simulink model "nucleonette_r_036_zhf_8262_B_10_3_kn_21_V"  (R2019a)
settings: Solver=VariableStepAuto  StartTime=0.0  StopTime=727544.216  FixedStep=0.2  RelTol=1e-6
libraries: simulink x6
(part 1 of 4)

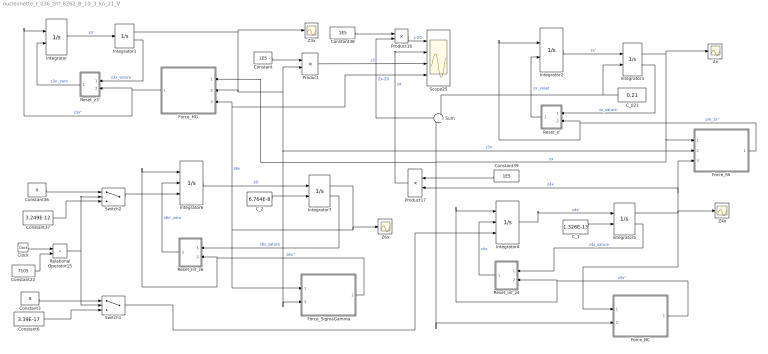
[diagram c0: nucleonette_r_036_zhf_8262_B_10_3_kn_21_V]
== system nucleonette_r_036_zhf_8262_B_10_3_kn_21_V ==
  C_021 : Constant  Value=0.21
  C_1 : Constant  Value=1.326E-13
  C_2 : Constant  Value=6.764E-8
  Clock : Clock
  Constant : Constant  Value=1E5
  Constant22 : Constant  Value=7105
  Constant3 : Constant  Value=0
  Constant36 : Constant  Value=0
  Constant37 : Constant  Value=3.249E-12
  Constant38 : Constant  Value=1E5
  Constant39 : Constant  Value=1E5
  Constant6 : Constant  Value=3.39E-17
  Force_BC : Subsystem
  Force_FA : Subsystem
  Force_HG : Subsystem
  Force_SigmaGamma : Subsystem
  Integrator : Integrator  ExternalReset=level
  Integrator1 : Integrator  LimitOutput=on  UpperSaturationLimit=0  LowerSaturationLimit=-1.80E-12  ShowSaturationPort=on  ZeroCross=off
  Integrator2 : Integrator  ExternalReset=level
  Integrator3 : Integrator  InitialConditionSource=external  LimitOutput=on  UpperSaturationLimit=0.21000000000316  LowerSaturationLimit=0.21  ShowSaturationPort=on
  Integrator4 : Integrator  ExternalReset=level  InitialConditionSource=external  AbsoluteTolerance=1E-22
  Integrator5 : Integrator  InitialConditionSource=external  LimitOutput=on  LowerSaturationLimit=0  ShowSaturationPort=on  ZeroCross=off
  Integrator6 : Integrator  ExternalReset=level  InitialConditionSource=external
  Integrator7 : Integrator  InitialConditionSource=external  LimitOutput=on  LowerSaturationLimit=0.0  ShowSaturationPort=on  ZeroCross=off
  Product : Product
  Product16 : Product
  Product17 : Product
  Relational Operator15 : RelationalOperator  Operator=>  OutDataTypeStr=boolean  RndMeth=Simplest
  Reset_Inf_z4 : Subsystem
  Reset_Inf_z6 : Subsystem
  Reset_z' : Subsystem
  Reset_z3' : Subsystem
  Scope25 : Scope  NumInputPorts=4
  Sum : Sum  Inputs=-+
  Switch1 : Switch  Criteria=u2 > Threshold
  Switch2 : Switch  Criteria=u2 > Threshold
  Z3x : Scope
  Z4x : Scope
  Z6x : Scope
  Zx : Scope
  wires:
  Integrator1/1 -> Z3x/1, Product/2, Force_FA/2(In2), Force_SigmaGamma/2(In2), Force_HG/2(In2)  "z3x"
  Integrator3/1 -> Force_HG/1(In1), Force_BC/2(In2), Sum/2, Force_FA/1(In1), Zx/1  "zx"
  C_021/1 -> Sum/1, Integrator3/2
  Force_FA/1(Out1) -> Integrator2/1, Reset_z'/2(In3)  "pre_zx''"
  Integrator3/2 -> Reset_z'/1(In1)  "zx_sature"
  Integrator2/1 -> Integrator3/1  "zx'"
  Force_HG/1(Out1) -> Integrator/1, Reset_z3'/2(In3)  "z3x''"
  Sum/1 -> Product16/2  "Zx-Z0"
  C_1/1 -> Integrator5/2
  Integrator5/2 -> Reset_Inf_z4/1(In1)  "z4x_sature"
  Integrator5/1 -> Product17/2, Force_FA/3(In3), Z4x/1, Force_BC/1(In1)  "z4x"
  Integrator7/2 -> Reset_Inf_z6/1(In1)  "z6x_sature"
  Reset_Inf_z6/1(Out1) -> Integrator6/2  "z6x'_zero"
  Integrator7/1 -> Z6x/1, Force_SigmaGamma/1(In1), Scope25/4, Force_HG/3(In3)  "z6x"
  Force_SigmaGamma/1(Out1) -> Reset_Inf_z6/2(In3), Integrator6/1  "z6x''"
  C_2/1 -> Integrator7/2
  Reset_z'/1(Out1) -> Integrator2/2  "zx'_reset"
  Integrator1/2 -> Reset_z3'/1(In1)  "z3x_sature"
  Reset_z3'/1(Out1) -> Integrator/2  "z3x'_zero"
  Integrator6/1 -> Integrator7/1  "z6'"
  Integrator4/1 -> Integrator5/1  "z4x'"
  Reset_Inf_z4/1(Out1) -> Integrator4/2  "z4x"
  Constant22/1 -> Relational Operator15/2
  Clock/1 -> Relational Operator15/1
  Constant6/1 -> Switch1/3
  Force_BC/1(Out1) -> Integrator4/1, Reset_Inf_z4/2(In3)  "z4x''"
  Switch1/1 -> Integrator4/3
  Constant3/1 -> Switch1/1
  Integrator/1 -> Integrator1/1  "z3'"
  Product/1 -> Scope25/3  "z3"
  Constant/1 -> Product/1
  Constant37/1 -> Switch2/3
  Constant36/1 -> Switch2/1
  Switch2/1 -> Integrator6/3
  Relational Operator15/1 -> Switch1/2, Switch2/2
  Product16/1 -> Scope25/1  "z-Z0"
  Constant38/1 -> Product16/1
  Constant39/1 -> Product17/1
  Product17/1 -> Scope25/2  "z4"

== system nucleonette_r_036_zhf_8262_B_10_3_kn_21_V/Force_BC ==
  In1 : Inport
  In2 : Inport  Port=2
  Add26 : Sum  Inputs=-++
  Constant23 : Constant  Value=3.16E-12
  F_BA : Subsystem
  F_BD : Subsystem
  F_BE : Subsystem
  F_BF : Subsystem
  F_CA : Subsystem
  F_CD : Subsystem
  F_CE : Subsystem
  F_CF : Subsystem
  Scope14 : Scope
  Sum1 : Sum  Inputs=|-|+|-|+|+|-|+|-
  Z0_1 : Constant  Value=0.21
  Out1 : Outport
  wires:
  Sum1/1 -> Scope14/1, Out1/1  "pre_z4x''"
  In1/1 -> F_CE/1(In1), F_BD/1(In1), F_CD/1(In1), F_CF/1(In1), F_CA/1(In1), F_BA/1(In1), F_BF/1(In1), F_BE/1(In1)  "z4"
  F_BF/1(Out1) -> Sum1/5
  F_BE/1(Out1) -> Sum1/1
  Z0_1/1 -> Add26/2  "Z0"
  In2/1 -> Add26/1  "z"
  Add26/1 -> F_CA/2(In2), F_BA/2(In2), F_CF/2(In2), F_BF/2(In2)  "z0 - z + delta"
  F_CE/1(Out1) -> Sum1/2
  F_BD/1(Out1) -> Sum1/3
  F_CD/1(Out1) -> Sum1/4
  F_CA/1(Out1) -> Sum1/8
  F_BA/1(Out1) -> Sum1/7
  Constant23/1 -> Add26/3  "Delta_1"
  F_CF/1(Out1) -> Sum1/6  "ncf/dcf_3"

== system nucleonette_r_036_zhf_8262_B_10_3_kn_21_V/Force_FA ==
  In1 : Inport
  In2 : Inport  Port=2
  In3 : Inport  Port=3
  Add1 : Sum  Inputs=-++
  Add26 : Sum  Inputs=-+
  Delta : Constant  Value=3.16E-12
  F_AB : Subsystem
  F_AC : Subsystem
  F_AD : Subsystem
  F_AE : Subsystem
  F_AG : Subsystem
  F_AH : Subsystem
  F_AI : Subsystem
  F_AJ : Subsystem
  F_FB : Subsystem
  F_FC : Subsystem
  F_FD : Subsystem
  F_FE : Subsystem
  F_FG : Subsystem
  F_FH : Subsystem
  F_FI : Subsystem
  F_FJ : Subsystem
  Scope1 : Scope
  Sum : Sum  Inputs=|++
  Sum1 : Sum  Inputs=|+|-|+|-|-|+|-|+
  Sum2 : Sum  Inputs=|-|+|+|-|-|+|+|-
  Z0_1 : Constant  Value=0.21
  Z0_2 : Constant  Value=0.21
  Out1 : Outport
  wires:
  Sum1/1 -> Sum/1  "pre_zx''_1"
  In1/1 -> F_AI/1(In1), F_AJ/1(In1), F_AG/1(In1), Add1/1, F_AH/1(In1), F_FH/1(In1), F_FG/1(In1), F_FJ/1(In1), F_FI/1(In1)
  F_FG/1(Out1) -> Sum1/5
  F_FI/1(Out1) -> Sum1/1
  Z0_1/1 -> Add26/2  "Z0"
  In2/1 -> Add26/1  "z3"
  Add26/1 -> F_FH/2(In2), F_AG/2(In2), F_FG/2(In2), F_AH/2(In2)  "z0 - z3"
  F_AI/1(Out1) -> Sum1/2
  F_FJ/1(Out1) -> Sum1/3
  F_AJ/1(Out1) -> Sum1/4
  F_AH/1(Out1) -> Sum1/8
  F_FH/1(Out1) -> Sum1/7
  F_AG/1(Out1) -> Sum1/6
  F_AE/1(Out1) -> Sum2/8
  F_FE/1(Out1) -> Sum2/7
  F_AD/1(Out1) -> Sum2/6
  Z0_2/1 -> Add1/2  "Z0"
  F_AC/1(Out1) -> Sum2/4
  F_FC/1(Out1) -> Sum2/3
  F_AB/1(Out1) -> Sum2/2
  Add1/1 -> F_AE/1(In1), F_FE/1(In1), F_AD/1(In1), F_FD/1(In1), F_AC/1(In1), F_FC/1(In1), F_AB/1(In1), F_FB/1(In1)  "z0 - z + delta"
  F_FB/1(Out1) -> Sum2/1
  F_FD/1(Out1) -> Sum2/5
  In3/1 -> F_AB/2(In2), F_FC/2(In2), F_AC/2(In2), F_FD/2(In2), F_AD/2(In2), F_AE/2(In2), F_FE/2(In2), F_FB/2(In2)
  Sum2/1 -> Sum/2  "pre_zx''_2"
  Sum/1 -> Scope1/1, Out1/1  "z3''"
  Delta/1 -> Add1/3  "Delta"

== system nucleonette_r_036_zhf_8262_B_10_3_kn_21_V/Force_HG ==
  In1 : Inport
  In2 : Inport  Port=2
  In3 : Inport  Port=3
  Add1 : Sum
  Add26 : Sum  Inputs=-+
  F_HA : Subsystem
  F_HF : Subsystem
  F_HGamma : Subsystem
  F_HI : Subsystem
  F_HJ : Subsystem
  F_HOmega : Subsystem
  F_HPhi : Subsystem
  F_HSigma : Subsystem
  Scope13 : Scope
  Sum : Sum  Inputs=|+|-|+|-
  Sum1 : Sum  Inputs=|+|+|-|-
  Sum2 : Sum  Inputs=|++
  Z0_1 : Constant  Value=0.21
  delta6 : Constant  Value=1.80E-12
  Out1 : Outport
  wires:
  In1/1 -> F_HJ/1(In1), F_HI/1(In1), F_HF/1(In1), F_HA/1(In1)  "zx"
  Sum/1 -> Sum2/1  "pre_z3x''_1"
  F_HA/1(Out1) -> Sum/1
  F_HF/1(Out1) -> Sum/2
  F_HI/1(Out1) -> Sum/3
  F_HJ/1(Out1) -> Sum/4
  F_HPhi/1(Out1) -> Sum1/3
  F_HOmega/1(Out1) -> Sum1/4
  F_HGamma/1(Out1) -> Sum1/2
  In3/1 -> F_HGamma/1(In1), F_HPhi/1(In1), F_HOmega/1(In1), F_HSigma/1(In1)  "z6x"
  F_HSigma/1(Out1) -> Sum1/1
  Sum1/1 -> Sum2/2  "pre_z3x''_2"
  Sum2/1 -> Scope13/1, Out1/1  "z3''"
  Z0_1/1 -> Add26/2  "Z0"
  In2/1 -> Add1/1, Add26/1  "Z3"
  Add26/1 -> F_HJ/2(In2), F_HI/2(In2), F_HF/2(In2), F_HA/2(In2)  "z0 - z3"
  Add1/1 -> F_HSigma/2(In2), F_HOmega/2(In2), F_HPhi/2(In2), F_HGamma/2(In2)  "z3 + delta6"
  delta6/1 -> Add1/2  "delta6"

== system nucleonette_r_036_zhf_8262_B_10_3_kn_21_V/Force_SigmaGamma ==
  In1 : Inport
  In2 : Inport  Port=2
  Add26 : Sum
  F_GammaG : Subsystem
  F_GammaH : Subsystem
  F_GammaOmega : Subsystem
  F_GammaPhi : Subsystem
  F_SigmaG : Subsystem
  F_SigmaH : Subsystem
  F_SigmaOmega : Subsystem
  F_SigmaPhi : Subsystem
  Scope14 : Scope
  Sum1 : Sum  Inputs=|+|-|+|-|+|-|+|-
  delta6 : Constant  Value=1.80E-12
  Out1 : Outport
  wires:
  Sum1/1 -> Scope14/1, Out1/1  "pre_z6x''"
  In1/1 -> F_SigmaOmega/1(In1), F_GammaOmega/1(In1), F_SigmaPhi/1(In1), F_GammaPhi/1(In1), F_SigmaH/1(In1), F_GammaH/1(In1), F_SigmaG/1(In1), F_GammaG/1(In1)  "z6"
  F_SigmaH/1(Out1) -> Sum1/5
  F_SigmaOmega/1(Out1) -> Sum1/1
  In2/1 -> Add26/1  "z3"
  Add26/1 -> F_GammaG/2(In2), F_SigmaG/2(In2), F_SigmaH/2(In2), F_GammaH/2(In2)  "delta6 + z3"
  F_GammaOmega/1(Out1) -> Sum1/2
  F_SigmaPhi/1(Out1) -> Sum1/3
  F_GammaPhi/1(Out1) -> Sum1/4
  F_GammaG/1(Out1) -> Sum1/8
  F_SigmaG/1(Out1) -> Sum1/7
  F_GammaH/1(Out1) -> Sum1/6
  delta6/1 -> Add26/2  "Delta6_1"

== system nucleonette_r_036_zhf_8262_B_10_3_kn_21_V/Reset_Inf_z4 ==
  In1 : Inport
  In3 : Inport  Port=2
  Compare To Zero : simulink/Logic and Bit Operations/Compare To Zero  relop=<  OutDataTypeStr=boolean
  Constant10 : Constant  Value=0
  Logical Operator1 : Logic  AllPortsSameDT=off  OutDataTypeStr=boolean
  Relational Operator4 : RelationalOperator  Operator=<  OutDataTypeStr=boolean  RndMeth=Simplest
  Out1 : Outport
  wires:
  In1/1 -> Compare To Zero/1  "Saturation"
  Constant10/1 -> Relational Operator4/2
  Compare To Zero/1 -> Logical Operator1/1
  Logical Operator1/1 -> Out1/1
  In3/1 -> Relational Operator4/1  "Acceleration"
  Relational Operator4/1 -> Logical Operator1/2  "ForceFz_>_0"

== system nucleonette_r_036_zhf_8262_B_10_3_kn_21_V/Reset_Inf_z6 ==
  In1 : Inport
  In3 : Inport  Port=2
  Compare To Zero : simulink/Logic and Bit Operations/Compare To Zero  relop=<  OutDataTypeStr=boolean
  Constant10 : Constant  Value=0
  Logical Operator1 : Logic  AllPortsSameDT=off  OutDataTypeStr=boolean
  Relational Operator4 : RelationalOperator  Operator=<  OutDataTypeStr=boolean  RndMeth=Simplest
  Out1 : Outport
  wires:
  In1/1 -> Compare To Zero/1  "Saturation"
  Constant10/1 -> Relational Operator4/2
  Compare To Zero/1 -> Logical Operator1/1
  Logical Operator1/1 -> Out1/1
  In3/1 -> Relational Operator4/1  "Acceleration"
  Relational Operator4/1 -> Logical Operator1/2  "ForceFz_>_0"

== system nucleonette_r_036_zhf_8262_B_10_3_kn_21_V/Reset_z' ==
  In1 : Inport
  In3 : Inport  Port=2
  Compare To Zero : simulink/Logic and Bit Operations/Compare To Zero  relop=>  OutDataTypeStr=boolean
  Compare To Zero1 : simulink/Logic and Bit Operations/Compare To Zero  relop=<  OutDataTypeStr=boolean
  Constant10 : Constant  Value=0
  Logical Operator1 : Logic  AllPortsSameDT=off  OutDataTypeStr=boolean
  Logical Operator2 : Logic  AllPortsSameDT=off  OutDataTypeStr=boolean
  Logical Operator3 : Logic  Operator=OR  AllPortsSameDT=off  OutDataTypeStr=boolean
  Relational Operator1 : RelationalOperator  Operator=<  OutDataTypeStr=boolean  RndMeth=Simplest
  Relational Operator4 : RelationalOperator  Operator=>  OutDataTypeStr=boolean  RndMeth=Simplest
  Out1 : Outport
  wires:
  In1/1 -> Compare To Zero1/1, Compare To Zero/1  "Saturation"
  Constant10/1 -> Relational Operator4/2, Relational Operator1/2
  Compare To Zero/1 -> Logical Operator1/1
  In3/1 -> Relational Operator1/1, Relational Operator4/1  "Acceleration"
  Relational Operator4/1 -> Logical Operator1/2  "Force_>_0"
  Compare To Zero1/1 -> Logical Operator2/2
  Relational Operator1/1 -> Logical Operator2/1  "Force_<_0"
  Logical Operator1/1 -> Logical Operator3/1
  Logical Operator2/1 -> Logical Operator3/2
  Logical Operator3/1 -> Out1/1

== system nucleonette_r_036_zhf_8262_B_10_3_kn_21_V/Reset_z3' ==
  In1 : Inport
  In3 : Inport  Port=2
  Compare To Zero : simulink/Logic and Bit Operations/Compare To Zero  relop=>  OutDataTypeStr=boolean
  Compare To Zero1 : simulink/Logic and Bit Operations/Compare To Zero  relop=<  OutDataTypeStr=boolean
  Constant10 : Constant  Value=0
  Logical Operator1 : Logic  AllPortsSameDT=off  OutDataTypeStr=boolean
  Logical Operator2 : Logic  AllPortsSameDT=off  OutDataTypeStr=boolean
  Logical Operator3 : Logic  Operator=OR  AllPortsSameDT=off  OutDataTypeStr=boolean
  Relational Operator1 : RelationalOperator  Operator=<  OutDataTypeStr=boolean  RndMeth=Simplest
  Relational Operator4 : RelationalOperator  Operator=>  OutDataTypeStr=boolean  RndMeth=Simplest
  Out1 : Outport
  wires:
  In1/1 -> Compare To Zero1/1, Compare To Zero/1  "Saturation"
  Constant10/1 -> Relational Operator4/2, Relational Operator1/2
  Compare To Zero/1 -> Logical Operator1/1
  In3/1 -> Relational Operator1/1, Relational Operator4/1  "Acceleration"
  Relational Operator4/1 -> Logical Operator1/2  "Force_>_0"
  Compare To Zero1/1 -> Logical Operator2/2
  Relational Operator1/1 -> Logical Operator2/1  "Force_<_0"
  Logical Operator1/1 -> Logical Operator3/1
  Logical Operator2/1 -> Logical Operator3/2
  Logical Operator3/1 -> Out1/1

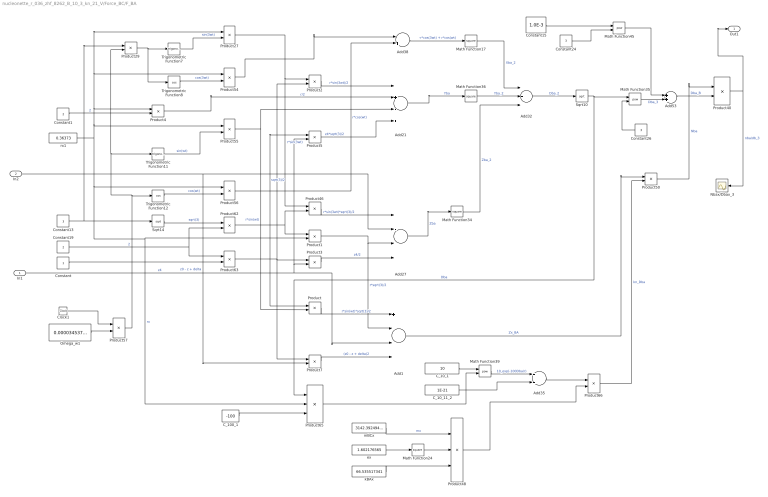
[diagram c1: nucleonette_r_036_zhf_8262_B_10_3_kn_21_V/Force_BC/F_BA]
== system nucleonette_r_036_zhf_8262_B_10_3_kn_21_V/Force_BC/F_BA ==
  In1 : Inport
  In2 : Inport  Port=2
  Add1 : Sum  Inputs=+---
  Add21 : Sum  Inputs=-+-+
  Add27 : Sum  Inputs=----
  Add32 : Sum  Inputs=+++
  Add35 : Sum
  Add38 : Sum  Inputs=-+
  Add53 : Sum
  C_100_1 : Constant  Value=-100
  C_10_1 : Constant  Value=10
  C_10_11_2 : Constant  Value=1E-21
  Clock1 : Clock
  Constant : Constant
  Constant1 : Constant  Value=2
  Constant13 : Constant  Value=3
  Constant15 : Constant  Value=1.0E-3
  Constant19 : Constant  Value=2
  Constant24 : Constant  Value=3
  Constant26 : Constant  Value=3
  Math Function{17,24,34,36} (4 alike) : Math  Operator=square
  Math Function35 : Math  Operator=pow
  Math Function39 : Math  Operator=pow
  Math Function45 : Math  Operator=pow
  Nbax/Dbax_3 : Scope
  Omega_w1 : Constant  Value=0.00003453723537
  Product{,1..3,5,7,29,46,50,57} (10 alike) : Product
  Product{27,54..56,66} (5 alike) : Product  Inputs=**
  Product4 : Product  Inputs=*/
  Product40 : Product  Inputs=*/
  Product48 : Product  Inputs=/**
  Product62 : Product  Inputs=*/
  Product63 : Product  Inputs=/*
  Product65 : Product  Inputs=*/*
  Sqrt10 : Sqrt
  Sqrt14 : Sqrt
  Trigonometric Function11 : Trigonometry
  Trigonometric Function12 : Trigonometry  Operator=cos
  Trigonometric Function7 : Trigonometry
  Trigonometric Function8 : Trigonometry  Operator=cos
  ex : Constant  Value=1.602176565
  kBAx : Constant  Value=66.535517341
  mBCx : Constant  Value=3142.392494946
  rx1 : Constant  Value=0.36373
  Out1 : Outport
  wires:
  Product/1 -> Add1/1  "r*sin(wt)*sqrt(3)/2"
  Product1/1 -> Add1/2, Add27/3  "r*sqrt(3)/2"
  Product63/1 -> Product7/1, Product2/2, Product3/1
  In1/1 -> Add1/3, Product5/2, Product3/2  "z4"
  Product3/1 -> Add27/4  "z4/2"
  Constant1/1 -> Product4/2  "2"
  Product5/1 -> Add21/4  "z4*sqrt(3)/2"
  Product4/1 -> Add21/2  "r/2"
  Add1/1 -> Product50/1  "Zx_BA"
  Product62/1 -> Product/1, Product1/1, Product46/2, Product5/1  "sqrt(3)/2"
  Product55/1 -> Add21/3, Product/2  "r*sin(wt)"
  Product40/1 -> Nbax/Dbax_3/1, Out1/1  "nba/db_3"
  Constant/1 -> Product63/2
  Add27/1 -> Math Function34/1  "Zba"
  Product50/1 -> Product40/1  "Nba"
  Trigonometric Function8/1 -> Product54/2  "cos(3wt)"
  Math Function35/1 -> Add53/2  "Dba_3"
  Clock1/1 -> Product57/1
  Omega_w1/1 -> Product57/2
  Product57/1 -> Product29/2, Trigonometric Function11/1, Trigonometric Function12/1
  Math Function45/1 -> Add53/1
  Product66/1 -> Product50/2  "kn_Dba"
  Constant15/1 -> Math Function45/1
  rx1/1 -> Product27/1, Product54/1, Product4/1, Product55/1, Product1/2, Product65/2, Product56/1  "rx"
  Math Function24/1 -> Product48/2
  Constant24/1 -> Math Function45/2
  Trigonometric Function11/1 -> Product55/2  "sin(wt)"
  Add35/1 -> Product66/1
  Product29/1 -> Trigonometric Function8/1, Trigonometric Function7/1
  Add21/1 -> Math Function36/1  "Yba"
  C_10_11_2/1 -> Add35/2
  Math Function34/1 -> Add32/3  "Zba_2"
  Constant13/1 -> Product29/1, Sqrt14/1
  kBAx/1 -> Product48/3
  Add32/1 -> Sqrt10/1  "Dba_2"
  Math Function39/1 -> Add35/1  "10_exp(-100Dba/r)"
  ex/1 -> Math Function24/1
  Product48/1 -> Product66/2
  Math Function17/1 -> Add32/1  "Xba_2"
  mBCx/1 -> Product48/1  "mx"
  Sqrt10/1 -> Product65/1, Math Function35/1  "Dba"
  Product54/1 -> Add38/1
  Product65/1 -> Math Function39/2
  Math Function36/1 -> Add32/2  "Yba_2"
  Constant26/1 -> Math Function35/2
  C_10_1/1 -> Math Function39/1
  C_100_1/1 -> Product65/3
  Add38/1 -> Math Function17/1  "-r*cos(3wt) + r*cos(wt)"
  Product2/1 -> Add21/1  "r*sin(3wt)/2"
  Sqrt14/1 -> Product62/1  "sqrt(3)"
  Constant19/1 -> Product63/1, Product62/2  "2"
  Trigonometric Function7/1 -> Product27/2  "sin(3wt)"
  Trigonometric Function12/1 -> Product56/2  "cos(wt)"
  Product56/1 -> Add38/2  "r*cos(wt)"
  In2/1 -> Add27/2, Product7/2  "z0 - z + delta"
  Product46/1 -> Add27/1  "r*sin(3wt)*sqrt(3)/2"
  Product27/1 -> Product2/1, Product46/1  "r*sin(3wt)"
  Add53/1 -> Product40/2  "Dba_B"
  Product7/1 -> Add1/4  "(z0 - z + delta)2"

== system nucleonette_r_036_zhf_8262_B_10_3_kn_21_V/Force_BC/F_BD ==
  In1 : Inport
  Add31 : Sum
  Add40 : Sum
  Add51 : Sum
  C_10 : Constant  Value=10
  C_100 : Constant  Value=-100
  C_10_11 : Constant  Value=1E-21
  Clock1 : Clock
  Constant : Constant  Value=3
  Constant1 : Constant  Value=2
  Constant15 : Constant  Value=1.0E-3
  Constant2 : Constant  Value=3
  Constant24 : Constant  Value=3
  Constant3 : Constant  Value=2
  Math Function27 : Math  Operator=square
  Math Function30 : Math  Operator=square
  Math Function32 : Math  Operator=pow
  Math Function37 : Math  Operator=pow
  Math Function4 : Math  Operator=square
  Math Function45 : Math  Operator=pow
  NBDx/DBDx_3 : Scope
  Omega_w1 : Constant  Value=0.00003453723537
  Product{1,4,6,12,45,57..58,60} (8 alike) : Product
  Product2 : Product  Inputs=*/
  Product26 : Product  Inputs=*/
  Product3 : Product  Inputs=/**
  Product31 : Product  Inputs=/**
  Product33 : Product  Inputs=/**
  Product44 : Product  Inputs=**
  Sqrt13 : Sqrt
  Sqrt4 : Sqrt
  Subtract3 : Sum  Inputs=+--
  Subtract4 : Sum
  Trigonometric Function9 : Trigonometry
  ex : Constant  Value=1.602176565
  keBDx : Constant  Value=598.819656066
  mBCx : Constant  Value=3142.392494946
  rx1 : Constant  Value=0.36373
  Out1 : Outport
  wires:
  Constant3/1 -> Product3/1
  Product2/1 -> Product6/1, Product12/2  "sqrt(3)/2"
  Product26/1 -> Out1/1, NBDx/DBDx_3/1  "F_BD"
  Product44/1 -> Subtract4/1  "z4*sqrt(3)"
  Constant1/1 -> Product2/2
  Add51/1 -> Product26/2  "DBD_B"
  ex/1 -> Math Function4/1
  Sqrt13/1 -> Product2/1, Product44/2, Product58/2  "sqrt(3)"
  Product6/1 -> Subtract3/2  "r*sqrt(3)/2"
  Subtract4/1 -> Math Function30/1  "YBD"
  Constant24/1 -> Math Function32/2, Math Function45/2
  Product3/1 -> Subtract3/3  "3z4/2"
  Math Function4/1 -> Product31/2
  Trigonometric Function9/1 -> Product4/1  "sin(3wt)"
  Clock1/1 -> Product57/1
  Product4/1 -> Product58/1, Product12/1  "r*sin(3wt)"
  In1/1 -> Product44/1, Product3/3  "z4"
  Product31/1 -> Product45/2
  C_10/1 -> Math Function37/1
  Constant/1 -> Sqrt13/1, Product1/2
  Product57/1 -> Product1/1  "angle_wt"
  Product1/1 -> Trigonometric Function9/1  "angle_3wt"
  Product60/1 -> Product26/1
  Subtract3/1 -> Product60/2  "Zx_BD"
  Constant2/1 -> Product3/2
  mBCx/1 -> Product31/1  "mx"
  Product33/1 -> Math Function37/2
  Sqrt4/1 -> Product33/2, Math Function32/1  "DBD"
  rx1/1 -> Product33/1, Subtract4/2, Product6/2, Product4/2  "rx"
  Math Function27/1 -> Add31/1  "ZBD_2"
  keBDx/1 -> Product31/3
  Omega_w1/1 -> Product57/2
  Constant15/1 -> Math Function45/1
  C_10_11/1 -> Add40/2
  Add31/1 -> Sqrt4/1
  Product58/1 -> Math Function27/1  "sqrt(3)*r*sin(3wt)"
  Product12/1 -> Subtract3/1  "r*sin(3wt)*sqrt(3)/2"
  Math Function30/1 -> Add31/2
  C_100/1 -> Product33/3
  Math Function37/1 -> Add40/1  "10_exp(-100Dbd/r)"
  Product45/1 -> Product60/1
  Math Function45/1 -> Add51/1
  Add40/1 -> Product45/1  "kn_DBD"
  Math Function32/1 -> Add51/2

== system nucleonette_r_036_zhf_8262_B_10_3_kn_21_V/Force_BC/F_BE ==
  In1 : Inport
  Add31 : Sum
  Add40 : Sum
  Add51 : Sum
  C_10 : Constant  Value=10
  C_100 : Constant  Value=-100
  C_10_11 : Constant  Value=1E-21
  Clock1 : Clock
  Constant : Constant  Value=3
  Constant1 : Constant  Value=2
  Constant15 : Constant  Value=1.0E-3
  Constant2 : Constant  Value=3
  Constant24 : Constant  Value=3
  Constant3 : Constant  Value=2
  Math Function27 : Math  Operator=square
  Math Function30 : Math  Operator=square
  Math Function32 : Math  Operator=pow
  Math Function37 : Math  Operator=pow
  Math Function4 : Math  Operator=square
  Math Function45 : Math  Operator=pow
  NBEx/DBEx_3 : Scope
  Omega_w1 : Constant  Value=0.00003453723537
  Product{1,4..6,12,45,57..58,60} (9 alike) : Product
  Product2 : Product  Inputs=*/
  Product26 : Product  Inputs=*/
  Product3 : Product  Inputs=/**
  Product31 : Product  Inputs=/**
  Product33 : Product  Inputs=/**
  Product44 : Product  Inputs=**
  Sqrt13 : Sqrt
  Sqrt4 : Sqrt
  Subtract3 : Sum  Inputs=-++
  Subtract4 : Sum  Inputs=++-
  Trigonometric Function10 : Trigonometry  Operator=cos
  Trigonometric Function9 : Trigonometry
  ex : Constant  Value=1.602176565
  keBEx : Constant  Value=598.819656066
  mBCx : Constant  Value=3142.392494946
  rx1 : Constant  Value=0.36373
  Out1 : Outport
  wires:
  Subtract4/1 -> Math Function30/1
  Math Function32/1 -> Add51/2
  Add40/1 -> Product45/1  "kn_DBE"
  Math Function45/1 -> Add51/1
  Product45/1 -> Product60/1
  Math Function4/1 -> Product31/2
  Math Function37/1 -> Add40/1  "10_exp(-100Dbe/r)"
  Clock1/1 -> Product57/1
  Subtract3/1 -> Product60/2  "ZBE"
  C_100/1 -> Product33/3
  Product58/1 -> Math Function27/1  "2r*cos(3wt)"
  Add51/1 -> Product26/2  "DBE_B"
  Add31/1 -> Sqrt4/1
  C_10_11/1 -> Add40/2
  Product31/1 -> Product45/2
  Product57/1 -> Product1/1  "angle_wt"
  C_10/1 -> Math Function37/1
  mBCx/1 -> Product31/1  "mx"
  Product33/1 -> Math Function37/2
  Constant15/1 -> Math Function45/1
  Omega_w1/1 -> Product57/2
  keBEx/1 -> Product31/3
  ex/1 -> Math Function4/1
  Math Function27/1 -> Add31/1  "XBE_2"
  Constant24/1 -> Math Function32/2, Math Function45/2
  rx1/1 -> Product33/1, Subtract4/2, Product5/2, Product6/2, Product4/2  "rx"
  Product26/1 -> Out1/1, NBEx/DBEx_3/1  "F_BE"
  Sqrt4/1 -> Product33/2, Math Function32/1  "DBE"
  In1/1 -> Product3/3, Product44/1  "z4"
  Product60/1 -> Product26/1
  Product1/1 -> Trigonometric Function10/1, Trigonometric Function9/1  "angle_3wt"
  Constant/1 -> Sqrt13/1, Product1/2
  Product44/1 -> Subtract4/1  "z4*sqrt(3)"
  Math Function30/1 -> Add31/2
  Product12/1 -> Subtract3/1  "r*sin(3wt)*sqrt(3)/2"
  Constant2/1 -> Product3/2
  Trigonometric Function9/1 -> Product4/1  "sin(3wt)"
  Trigonometric Function10/1 -> Product5/1  "cos(3wt)"
  Product4/1 -> Subtract4/3, Product12/1  "r*sin(3wt)"
  Product3/1 -> Subtract3/3  "3z4/2"
  Product6/1 -> Subtract3/2  "r*sqrt(3)/2"
  Product5/1 -> Product58/2  "r*cos(3wt)"
  Sqrt13/1 -> Product2/1, Product44/2  "sqrt(3)"
  Constant1/1 -> Product2/2
  Product2/1 -> Product6/1, Product12/2  "sqrt(3)/2"
  Constant3/1 -> Product58/1, Product3/1

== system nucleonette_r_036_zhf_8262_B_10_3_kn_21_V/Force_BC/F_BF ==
  In1 : Inport
  In2 : Inport  Port=2
  Add1 : Sum  Inputs=++++
  Add21 : Sum  Inputs=+---
  Add27 : Sum  Inputs=++++
  Add32 : Sum  Inputs=+++
  Add35 : Sum
  Add38 : Sum
  Add53 : Sum
  C_100_1 : Constant  Value=-100
  C_10_1 : Constant  Value=10
  C_10_11_2 : Constant  Value=1E-21
  Clock1 : Clock
  Constant : Constant
  Constant1 : Constant  Value=2
  Constant13 : Constant  Value=3
  Constant15 : Constant  Value=1.0E-3
  Constant19 : Constant  Value=2
  Constant24 : Constant  Value=3
  Constant26 : Constant  Value=3
  Math Function{17,24,34,36} (4 alike) : Math  Operator=square
  Math Function35 : Math  Operator=pow
  Math Function39 : Math  Operator=pow
  Math Function45 : Math  Operator=pow
  Nbfx/Dbfx_3 : Scope
  Omega_w1 : Constant  Value=0.00003453723537
  Product{,1..3,5,7,29,46,50,57} (10 alike) : Product
  Product{27,54..56,66} (5 alike) : Product  Inputs=**
  Product4 : Product  Inputs=*/
  Product40 : Product  Inputs=*/
  Product48 : Product  Inputs=/**
  Product62 : Product  Inputs=*/
  Product63 : Product  Inputs=/*
  Product65 : Product  Inputs=*/*
  Sqrt10 : Sqrt
  Sqrt14 : Sqrt
  Trigonometric Function11 : Trigonometry
  Trigonometric Function12 : Trigonometry  Operator=cos
  Trigonometric Function7 : Trigonometry
  Trigonometric Function8 : Trigonometry  Operator=cos
  ex : Constant  Value=1.602176565
  kBFx : Constant  Value=66.535517341
  mBCx : Constant  Value=3142.392494946
  rx1 : Constant  Value=0.36373
  Out1 : Outport
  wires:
  Product50/1 -> Product40/1  "Nbf"
  C_10_1/1 -> Math Function39/1
  Constant26/1 -> Math Function35/2
  Product27/1 -> Product2/1, Product46/1  "r*sin(3wt)"
  Product46/1 -> Add27/1  "r*sin(3wt)*sqrt(3)/2"
  Product65/1 -> Math Function39/2
  Math Function36/1 -> Add32/2  "Ybf_2"
  Sqrt10/1 -> Product65/1, Math Function35/1  "Dbf"
  Math Function24/1 -> Product48/2
  mBCx/1 -> Product48/1  "mx"
  Math Function17/1 -> Add32/1  "Xbf_2"
  ex/1 -> Math Function24/1
  kBFx/1 -> Product48/3
  Add53/1 -> Product40/2  "Dbf_B"
  Add27/1 -> Math Function34/1  "Zbf"
  C_100_1/1 -> Product65/3
  Add38/1 -> Math Function17/1  "r*cos(3wt) + r*cos(wt)"
  Add32/1 -> Sqrt10/1  "Dbf_2"
  Constant13/1 -> Product29/1, Sqrt14/1
  Constant15/1 -> Math Function45/1
  Add35/1 -> Product66/1
  Math Function34/1 -> Add32/3  "Zbf_2"
  Product29/1 -> Trigonometric Function8/1, Trigonometric Function7/1
  Add21/1 -> Math Function36/1  "Ybf"
  Constant24/1 -> Math Function45/2
  Trigonometric Function11/1 -> Product55/2  "sin(wt)"
  Trigonometric Function8/1 -> Product54/2  "cos(3wt)"
  Trigonometric Function12/1 -> Product56/2  "cos(wt)"
  rx1/1 -> Product27/1, Product54/1, Product4/1, Product55/1, Product1/2, Product65/2, Product56/1  "rx"
  Trigonometric Function7/1 -> Product27/2  "sin(3wt)"
  Math Function39/1 -> Add35/1  "10_exp(-100Dbf/r)"
  Product48/1 -> Product66/2
  C_10_11_2/1 -> Add35/2
  Math Function35/1 -> Add53/2  "Dbf_3"
  Product66/1 -> Product50/2  "kn_Dbf"
  Math Function45/1 -> Add53/1
  Clock1/1 -> Product57/1
  Product57/1 -> Product29/2, Trigonometric Function11/1, Trigonometric Function12/1
  Omega_w1/1 -> Product57/2
  Product40/1 -> Nbfx/Dbfx_3/1, Out1/1  "nbf/dbf_3"
  In2/1 -> Add27/2, Product7/2  "z0 - z + delta"
  Sqrt14/1 -> Product62/1  "sqrt(3)"
  Constant19/1 -> Product63/1, Product62/2  "2"
  Product62/1 -> Product/1, Product1/1, Product46/2, Product5/1  "sqrt(3)/2"
  Product1/1 -> Add1/2, Add27/3  "r*sqrt(3)/2"
  Product56/1 -> Add38/2  "r*cos(wt)"
  Product54/1 -> Add38/1
  Product63/1 -> Product7/1, Product2/2, Product3/1
  In1/1 -> Add1/3, Product5/2, Product3/2  "z4"
  Product3/1 -> Add27/4  "z4/2"
  Constant/1 -> Product63/2
  Product2/1 -> Add21/1  "r*sin(3wt)/2"
  Product5/1 -> Add21/4  "z4*sqrt(3)/2"
  Product55/1 -> Add21/3, Product/2  "r*sin(wt)"
  Product4/1 -> Add21/2  "r/2"
  Constant1/1 -> Product4/2  "2"
  Product/1 -> Add1/1
  Add1/1 -> Product50/1  "Zx_BF"
  Product7/1 -> Add1/4  "(z0 - z + delta)2"

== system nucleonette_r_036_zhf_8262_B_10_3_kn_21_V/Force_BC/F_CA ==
  In1 : Inport
  In2 : Inport  Port=2
  Add1 : Sum  Inputs=+---
  Add21 : Sum  Inputs=--+-
  Add27 : Sum  Inputs=-+++
  Add32 : Sum  Inputs=+++
  Add35 : Sum
  Add38 : Sum  Inputs=--
  Add53 : Sum
  C_100_1 : Constant  Value=-100
  C_10_1 : Constant  Value=10
  C_10_11_2 : Constant  Value=1E-21
  Clock1 : Clock
  Constant : Constant
  Constant1 : Constant  Value=2
  Constant13 : Constant  Value=3
  Constant15 : Constant  Value=1.0E-3
  Constant19 : Constant  Value=2
  Constant24 : Constant  Value=3
  Constant26 : Constant  Value=3
  Math Function{17,24,34,36} (4 alike) : Math  Operator=square
  Math Function35 : Math  Operator=pow
  Math Function39 : Math  Operator=pow
  Math Function45 : Math  Operator=pow
  Ncax/Dcax_3 : Scope
  Omega_w1 : Constant  Value=0.00003453723537
  Product{,1..3,5,7,29,46,50,57} (10 alike) : Product
  Product{27,54..56,66} (5 alike) : Product  Inputs=**
  Product4 : Product  Inputs=*/
  Product40 : Product  Inputs=*/
  Product48 : Product  Inputs=/**
  Product62 : Product  Inputs=*/
  Product63 : Product  Inputs=/*
  Product65 : Product  Inputs=*/*
  Sqrt10 : Sqrt
  Sqrt14 : Sqrt
  Trigonometric Function11 : Trigonometry
  Trigonometric Function12 : Trigonometry  Operator=cos
  Trigonometric Function7 : Trigonometry
  Trigonometric Function8 : Trigonometry  Operator=cos
  ex : Constant  Value=1.602176565
  kBAx : Constant  Value=66.535517341
  mBCx : Constant  Value=3142.392494946
  rx1 : Constant  Value=0.36373
  Out1 : Outport
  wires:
  Constant24/1 -> Math Function45/2
  Add53/1 -> Product40/2  "Dca_B"
  Product27/1 -> Product2/1, Product46/1  "r*sin(3wt)"
  Product56/1 -> Add38/2  "r*cos(wt)"
  In2/1 -> Add27/2, Product7/2  "z0 - z + delta"
  Product29/1 -> Trigonometric Function8/1, Trigonometric Function7/1
  Add32/1 -> Sqrt10/1  "Dca_2"
  Trigonometric Function12/1 -> Product56/2  "cos(wt)"
  Constant26/1 -> Math Function35/2
  Product50/1 -> Product40/1  "Nca"
  Trigonometric Function7/1 -> Product27/2  "sin(3wt)"
  Product40/1 -> Ncax/Dcax_3/1, Out1/1  "nca/ca_3"
  Math Function35/1 -> Add53/2  "Dca_3"
  C_10_1/1 -> Math Function39/1
  Constant19/1 -> Product63/1, Product62/2  "2"
  Sqrt14/1 -> Product62/1  "sqrt(3)"
  Product62/1 -> Product/1, Product1/1, Product46/2, Product5/1  "sqrt(3)/2"
  Product2/1 -> Add21/1  "r*sin(3wt)/2"
  kBAx/1 -> Product48/3
  Add38/1 -> Math Function17/1  "-r*cos(3wt) - r*cos(wt)"
  Product/1 -> Add1/1  "r*sin(wt)*sqrt(3)/2"
  mBCx/1 -> Product48/1  "mx"
  Product48/1 -> Product66/2
  Product65/1 -> Math Function39/2
  Product54/1 -> Add38/1
  Sqrt10/1 -> Product65/1, Math Function35/1  "Dca"
  Math Function24/1 -> Product48/2
  Math Function17/1 -> Add32/1  "Xca_2"
  Constant13/1 -> Product29/1, Sqrt14/1
  Constant1/1 -> Product4/2  "2"
  ex/1 -> Math Function24/1
  Omega_w1/1 -> Product57/2
  Constant/1 -> Product63/2
  Math Function39/1 -> Add35/1  "10_exp(-100Dca/r)"
  Add27/1 -> Math Function34/1  "Zca"
  Clock1/1 -> Product57/1
  Math Function34/1 -> Add32/3  "Zca_2"
  Add21/1 -> Math Function36/1  "Yca"
  Product46/1 -> Add27/1  "r*sin(3wt)*sqrt(3)/2"
  Math Function45/1 -> Add53/1
  C_10_11_2/1 -> Add35/2
  Math Function36/1 -> Add32/2  "Yca_2"
  Constant15/1 -> Math Function45/1
  Product66/1 -> Product50/2  "kn_Dca"
  Product57/1 -> Product29/2, Trigonometric Function11/1, Trigonometric Function12/1  "angle_wt"
  Trigonometric Function8/1 -> Product54/2  "cos(3wt)"
  Product5/1 -> Add21/4  "z4*sqrt(3)/2"
  Product55/1 -> Add21/3, Product/2  "r*sin(wt)"
  Add1/1 -> Product50/1  "Zx_CA"
  Product4/1 -> Add21/2  "r/2"
  Product3/1 -> Add27/4  "z4/2"
  In1/1 -> Add1/3, Product5/2, Product3/2  "z4"
  Trigonometric Function11/1 -> Product55/2  "sin(wt)"
  C_100_1/1 -> Product65/3
  Product1/1 -> Add1/2, Add27/3  "r*sqrt(3)/2"
  rx1/1 -> Product27/1, Product54/1, Product4/1, Product55/1, Product1/2, Product65/2, Product56/1  "rx"
  Add35/1 -> Product66/1
  Product63/1 -> Product7/1, Product2/2, Product3/1
  Product7/1 -> Add1/4  "(z0 - z + delta)2"

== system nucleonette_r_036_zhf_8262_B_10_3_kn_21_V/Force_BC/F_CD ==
  In1 : Inport
  Add31 : Sum
  Add40 : Sum
  Add51 : Sum
  C_10 : Constant  Value=10
  C_100 : Constant  Value=-100
  C_10_11 : Constant  Value=1E-21
  Clock1 : Clock
  Constant : Constant  Value=3
  Constant1 : Constant  Value=2
  Constant15 : Constant  Value=1.0E-3
  Constant17 : Constant  Value=-1E-17
  Constant2 : Constant  Value=3
  Constant24 : Constant  Value=3
  Constant3 : Constant  Value=2
  Math Function27 : Math  Operator=square
  Math Function30 : Math  Operator=square
  Math Function32 : Math  Operator=pow
  Math Function37 : Math  Operator=pow
  Math Function4 : Math  Operator=square
  Math Function45 : Math  Operator=pow
  NCDx/DCDx_1 : Scope
  NCDx/DCDx_3 : Scope
  Omega_w1 : Constant  Value=0.00003453723537
  Product{1,4..6,12,45,57..58,60,75} (10 alike) : Product
  Product2 : Product  Inputs=*/
  Product26 : Product  Inputs=*/
  Product3 : Product  Inputs=/**
  Product31 : Product  Inputs=/**
  Product33 : Product  Inputs=/**
  Product44 : Product  Inputs=**
  Relational Operator1 : RelationalOperator  Operator=<  OutDataTypeStr=boolean  RndMeth=Simplest
  Sqrt13 : Sqrt
  Sqrt4 : Sqrt
  Subtract3 : Sum  Inputs=---
  Subtract4 : Sum  Inputs=+++
  Trigonometric Function10 : Trigonometry  Operator=cos
  Trigonometric Function9 : Trigonometry
  ex : Constant  Value=1.602176565
  keCDx : Constant  Value=598.819656066
  mBCx : Constant  Value=3142.392494946
  rx1 : Constant  Value=0.36373
  Out1 : Outport
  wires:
  Constant3/1 -> Product3/1, Product58/1
  Product2/1 -> Product6/1, Product12/2  "sqrt(3)/2"
  In1/1 -> Product44/1, Product3/3  "z4"
  Product26/1 -> Out1/1, Product75/2, Relational Operator1/2, NCDx/DCDx_3/1  "F_CD"
  Product44/1 -> Subtract4/1  "z4*sqrt(3)"
  Constant1/1 -> Product2/2
  Add51/1 -> Product26/2  "DCD_B"
  ex/1 -> Math Function4/1
  Sqrt13/1 -> Product2/1, Product44/2  "sqrt(3)"
  Product6/1 -> Subtract3/2  "r*sqrt(3)/2"
  Subtract4/1 -> Math Function30/1  "YCD"
  Constant24/1 -> Math Function32/2, Math Function45/2
  Product3/1 -> Subtract3/3  "3z4/2"
  Math Function4/1 -> Product31/2
  Trigonometric Function9/1 -> Product4/1  "sin(3wt)"
  Clock1/1 -> Product57/1
  Product4/1 -> Subtract4/3, Product12/1  "r*sin(3wt)"
  Product31/1 -> Product45/2
  C_10/1 -> Math Function37/1
  Constant/1 -> Sqrt13/1, Product1/2
  Product1/1 -> Trigonometric Function10/1, Trigonometric Function9/1  "angle_3wt"
  Product57/1 -> Product1/1  "angle_wt"
  Product60/1 -> Product26/1
  Subtract3/1 -> Product60/2  "Zx_CD"
  Constant2/1 -> Product3/2
  Trigonometric Function10/1 -> Product5/1  "cos(3wt)"
  mBCx/1 -> Product31/1  "mx"
  Product33/1 -> Math Function37/2
  Relational Operator1/1 -> Product75/1
  Sqrt4/1 -> Product33/2, Math Function32/1  "DCD"
  rx1/1 -> Product33/1, Product5/2, Product6/2, Product4/2, Subtract4/2  "rx"
  Math Function27/1 -> Add31/1  "ZCD_2"
  Product75/1 -> NCDx/DCDx_1/1  "FCD_1"
  keCDx/1 -> Product31/3
  Omega_w1/1 -> Product57/2
  C_10_11/1 -> Add40/2
  Constant15/1 -> Math Function45/1
  Add31/1 -> Sqrt4/1
  Product58/1 -> Math Function27/1  "2*r*cos(3wt)"
  Product12/1 -> Subtract3/1  "r*sin(3wt)*sqrt(3)/2"
  Math Function30/1 -> Add31/2
  Constant17/1 -> Relational Operator1/1
  C_100/1 -> Product33/3
  Math Function37/1 -> Add40/1  "10_exp(-100Dcd/r)"
  Product45/1 -> Product60/1
  Math Function45/1 -> Add51/1
  Math Function32/1 -> Add51/2
  Add40/1 -> Product45/1  "kn_DCD"
  Product5/1 -> Product58/2  "r*cos(3wt)"

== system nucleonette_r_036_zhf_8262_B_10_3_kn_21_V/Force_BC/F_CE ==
  In1 : Inport
  Add31 : Sum
  Add40 : Sum
  Add51 : Sum
  C_10 : Constant  Value=10
  C_100 : Constant  Value=-100
  C_10_11 : Constant  Value=1E-21
  Clock1 : Clock
  Constant : Constant  Value=3
  Constant1 : Constant  Value=2
  Constant15 : Constant  Value=1.0E-3
  Constant2 : Constant  Value=3
  Constant24 : Constant  Value=3
  Constant3 : Constant  Value=2
  Math Function27 : Math  Operator=square
  Math Function30 : Math  Operator=square
  Math Function32 : Math  Operator=pow
  Math Function37 : Math  Operator=pow
  Math Function4 : Math  Operator=square
  Math Function45 : Math  Operator=pow
  NCEx/DCEx_3 : Scope
  Omega_w1 : Constant  Value=0.00003453723537
  Product{1,4,6,12,45,57..58,60} (8 alike) : Product
  Product2 : Product  Inputs=*/
  Product26 : Product  Inputs=*/
  Product3 : Product  Inputs=/**
  Product31 : Product  Inputs=/**
  Product33 : Product  Inputs=/**
  Product44 : Product  Inputs=**
  Sqrt13 : Sqrt
  Sqrt4 : Sqrt
  Subtract3 : Sum  Inputs=-++
  Subtract4 : Sum
  Trigonometric Function9 : Trigonometry
  ex : Constant  Value=1.602176565
  keCEx : Constant  Value=598.819656066
  mBCx : Constant  Value=3142.392494946
  rx1 : Constant  Value=0.36373
  Out1 : Outport
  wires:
  Constant3/1 -> Product3/1
  Product2/1 -> Product6/1, Product12/2  "sqrt(3)/2"
  In1/1 -> Product44/1, Product3/3  "z4"
  Product26/1 -> Out1/1, NCEx/DCEx_3/1  "F_CE"
  Product44/1 -> Subtract4/1  "z4*sqrt(3)"
  Constant1/1 -> Product2/2
  Add51/1 -> Product26/2  "DCE_B"
  ex/1 -> Math Function4/1
  Sqrt13/1 -> Product2/1, Product44/2, Product58/2  "sqrt(3)"
  Product6/1 -> Subtract3/2  "r*sqrt(3)/2"
  Subtract4/1 -> Math Function30/1  "YCE"
  Constant24/1 -> Math Function32/2, Math Function45/2
  Product3/1 -> Subtract3/3  "3z4/2"
  Math Function4/1 -> Product31/2
  Trigonometric Function9/1 -> Product4/1  "sin(3wt)"
  Clock1/1 -> Product57/1
  Product4/1 -> Product58/1, Product12/1  "r*sin(3wt)"
  Product31/1 -> Product45/2
  C_10/1 -> Math Function37/1
  Constant/1 -> Sqrt13/1, Product1/2
  Product1/1 -> Trigonometric Function9/1  "angle_3wt"
  Product57/1 -> Product1/1  "angle_wt"
  Product60/1 -> Product26/1
  Subtract3/1 -> Product60/2  "Zx_CE"
  Constant2/1 -> Product3/2
  mBCx/1 -> Product31/1  "mx"
  Product33/1 -> Math Function37/2
  Sqrt4/1 -> Product33/2, Math Function32/1  "DCE"
  rx1/1 -> Product33/1, Subtract4/2, Product6/2, Product4/2  "rx"
  Math Function27/1 -> Add31/1  "ZCE_2"
  keCEx/1 -> Product31/3
  Omega_w1/1 -> Product57/2
  C_10_11/1 -> Add40/2
  Constant15/1 -> Math Function45/1
  Add31/1 -> Sqrt4/1
  Product58/1 -> Math Function27/1  "sqrt(3)*r*sin(3wt)"
  Product12/1 -> Subtract3/1  "r*sin(3wt)*sqrt(3)/2"
  Math Function30/1 -> Add31/2
  C_100/1 -> Product33/3
  Math Function37/1 -> Add40/1  "10_exp(-100Dce/r)"
  Product45/1 -> Product60/1
  Math Function45/1 -> Add51/1
  Math Function32/1 -> Add51/2
  Add40/1 -> Product45/1  "kn_DCE"

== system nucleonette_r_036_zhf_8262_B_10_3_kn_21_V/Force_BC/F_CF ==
  In1 : Inport
  In2 : Inport  Port=2
  Add1 : Sum  Inputs=++++
  Add21 : Sum  Inputs=----
  Add27 : Sum  Inputs=-+++
  Add32 : Sum  Inputs=+++
  Add35 : Sum
  Add38 : Sum  Inputs=-+
  Add53 : Sum
  C_100_1 : Constant  Value=-100
  C_10_1 : Constant  Value=10
  C_10_11_2 : Constant  Value=1E-21
  Clock1 : Clock
  Constant : Constant
  Constant1 : Constant  Value=2
  Constant13 : Constant  Value=3
  Constant15 : Constant  Value=1.0E-3
  Constant19 : Constant  Value=2
  Constant24 : Constant  Value=3
  Constant26 : Constant  Value=3
  Math Function{17,24,34,36} (4 alike) : Math  Operator=square
  Math Function35 : Math  Operator=pow
  Math Function39 : Math  Operator=pow
  Math Function45 : Math  Operator=pow
  Nbcx/Dcfx_3 : Scope
  Omega_w1 : Constant  Value=0.00003453723537
  Product{,1..3,5,7,29,46,50,57} (10 alike) : Product
  Product{27,54..56,66} (5 alike) : Product  Inputs=**
  Product4 : Product  Inputs=*/
  Product40 : Product  Inputs=*/
  Product48 : Product  Inputs=/**
  Product62 : Product  Inputs=*/
  Product63 : Product  Inputs=/*
  Product65 : Product  Inputs=*/*
  Sqrt10 : Sqrt
  Sqrt14 : Sqrt
  Trigonometric Function11 : Trigonometry
  Trigonometric Function12 : Trigonometry  Operator=cos
  Trigonometric Function7 : Trigonometry
  Trigonometric Function8 : Trigonometry  Operator=cos
  ex : Constant  Value=1.602176565
  kCFx : Constant  Value=66.535517341
  mBCx : Constant  Value=3142.392494946
  rx1 : Constant  Value=0.36373
  Out1 : Outport
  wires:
  Add1/1 -> Product50/1  "Zx_CF"
  Math Function34/1 -> Add32/3  "Zcf_2"
  Product48/1 -> Product66/2
  Product3/1 -> Add27/4  "z4/2"
  Product4/1 -> Add21/2  "r/2"
  Product/1 -> Add1/1
  Constant13/1 -> Product29/1, Sqrt14/1
  Add38/1 -> Math Function17/1  "-r*cos(3wt) + r*cos(wt)"
  Math Function24/1 -> Product48/2
  Trigonometric Function7/1 -> Product27/2  "sin(3wt)"
  Add35/1 -> Product66/1
  Product2/1 -> Add21/1  "r*sin(3wt)/2"
  Constant/1 -> Product63/2
  Product54/1 -> Add38/1
  Product56/1 -> Add38/2  "r*cos(wt)"
  C_10_11_2/1 -> Add35/2
  Product1/1 -> Add1/2, Add27/3  "r*sqrt(3)/2"
  Product62/1 -> Product/1, Product1/1, Product46/2, Product5/1  "sqrt(3)/2"
  Product40/1 -> Nbcx/Dcfx_3/1, Out1/1  "ncf/dcf_3"
  Constant19/1 -> Product63/1, Product62/2  "2"
  Add53/1 -> Product40/2  "Dcf_B"
  Sqrt14/1 -> Product62/1  "sqrt(3)"
  Sqrt10/1 -> Product65/1, Math Function35/1  "Dcf"
  Product63/1 -> Product7/1, Product2/2, Product3/1
  Add32/1 -> Sqrt10/1  "Dcf_2"
  In1/1 -> Add1/3, Product5/2, Product3/2  "z4"
  In2/1 -> Add27/2, Product7/2  "z0 - z + delta"
  Product57/1 -> Product29/2, Trigonometric Function11/1, Trigonometric Function12/1
  C_10_1/1 -> Math Function39/1
  Math Function39/1 -> Add35/1  "10_exp(-100Dcf/r)"
  Math Function45/1 -> Add53/1
  mBCx/1 -> Product48/1  "mx"
  Omega_w1/1 -> Product57/2
  Product66/1 -> Product50/2  "kn_Dcf"
  Product55/1 -> Add21/3, Product/2  "r*sin(wt)"
  Trigonometric Function8/1 -> Product54/2  "cos(3wt)"
  Trigonometric Function12/1 -> Product56/2  "cos(wt)"
  Trigonometric Function11/1 -> Product55/2  "sin(wt)"
  Math Function36/1 -> Add32/2  "Ycf_2"
  Constant24/1 -> Math Function45/2
  Constant15/1 -> Math Function45/1
  Add21/1 -> Math Function36/1  "Ycf"
  Product29/1 -> Trigonometric Function8/1, Trigonometric Function7/1
  C_100_1/1 -> Product65/3
  Clock1/1 -> Product57/1
  Add27/1 -> Math Function34/1  "Zcf"
  Product5/1 -> Add21/4  "z4*sqrt(3)/2"
  rx1/1 -> Product27/1, Product54/1, Product4/1, Product55/1, Product1/2, Product65/2, Product56/1  "rx"
  kCFx/1 -> Product48/3
  ex/1 -> Math Function24/1
  Math Function17/1 -> Add32/1  "Xcf_2"
  Product65/1 -> Math Function39/2
  Math Function35/1 -> Add53/2  "Dcf_3"
  Product46/1 -> Add27/1  "r*sin(3wt)*sqrt(3)/2"
  Constant1/1 -> Product4/2  "2"
  Product50/1 -> Product40/1  "Ncf"
  Product27/1 -> Product2/1, Product46/1  "r*sin(3wt)"
  Constant26/1 -> Math Function35/2
  Product7/1 -> Add1/4  "(z0 - z + delta)2"

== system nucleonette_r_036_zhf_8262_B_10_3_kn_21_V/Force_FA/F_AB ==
  In1 : Inport
  In2 : Inport  Port=2
  Add21 : Sum  Inputs=+-
  Add27 : Sum  Inputs=++++
  Add32 : Sum  Inputs=+++
  Add35 : Sum
  Add38 : Sum  Inputs=+--+
  Add53 : Sum
  C_100_1 : Constant  Value=-100
  C_10_1 : Constant  Value=10
  C_10_11_2 : Constant  Value=1E-21
  Clock1 : Clock
  Constant : Constant
  Constant1 : Constant  Value=2
  Constant13 : Constant  Value=3
  Constant15 : Constant  Value=1.0E-3
  Constant19 : Constant  Value=2
  Constant24 : Constant  Value=3
  Constant26 : Constant  Value=3
  Math Function{17,24,34,36} (4 alike) : Math  Operator=square
  Math Function35 : Math  Operator=pow
  Math Function39 : Math  Operator=pow
  Math Function45 : Math  Operator=pow
  Nabx/Dabx : Scope
  Omega_w1 : Constant  Value=0.00003453723537
  Product{1..4,27,54..56,66} (9 alike) : Product  Inputs=**
  Product{29,46,50,57} (4 alike) : Product
  Product40 : Product  Inputs=*/
  Product48 : Product  Inputs=/**
  Product5 : Product  Inputs=/*
  Product62 : Product  Inputs=*/
  Product63 : Product  Inputs=/*
  Product65 : Product  Inputs=*/*
  Sqrt10 : Sqrt
  Sqrt14 : Sqrt
  Trigonometric Function11 : Trigonometry
  Trigonometric Function12 : Trigonometry  Operator=cos
  Trigonometric Function7 : Trigonometry
  Trigonometric Function8 : Trigonometry  Operator=cos
  ex : Constant  Value=1.602176565
  kABx : Constant  Value=66.535517341
  mFAx : Constant  Value=999.755388642
  rx1 : Constant  Value=0.36373
  Out1 : Outport
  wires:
  Product2/1 -> Add38/3  "z4*sqrt(3)/2"
  In2/1 -> Product1/1  "z4"
  Product56/1 -> Add21/2  "r*cos(wt)"
  C_10_1/1 -> Math Function39/1
  Math Function34/1 -> Add32/3  "Zab_2"
  Clock1/1 -> Product57/1
  Trigonometric Function12/1 -> Product56/2  "cos(wt)"
  Constant26/1 -> Math Function35/2
  Product46/1 -> Add27/1  "r*sin(3wt)*sqrt(3)/2"
  Product65/1 -> Math Function39/2
  Constant15/1 -> Math Function45/1
  C_100_1/1 -> Product65/3
  Math Function36/1 -> Add32/2  "Xab_2"
  mFAx/1 -> Product48/1  "mx"
  Add38/1 -> Math Function17/1  "YAB"
  Sqrt10/1 -> Product65/1, Math Function35/1  "Dab"
  C_10_11_2/1 -> Add35/2
  Math Function17/1 -> Add32/1  "Yab_2"
  Add53/1 -> Product40/2  "Dab_B"
  kABx/1 -> Product48/3
  Product66/1 -> Product50/2  "kn_Dab"
  Product29/1 -> Trigonometric Function8/1, Trigonometric Function7/1
  Product27/1 -> Product46/1, Product62/1  "r*sin(3wt)"
  Add32/1 -> Sqrt10/1  "Dab_2"
  Product40/1 -> Nabx/Dabx/1, Out1/1  "nab/dab"
  Omega_w1/1 -> Product57/2
  Constant13/1 -> Product29/1, Sqrt14/1
  Add35/1 -> Product66/1
  Add21/1 -> Math Function36/1  "XAB"
  Trigonometric Function11/1 -> Product55/2  "sin(wt)"
  Trigonometric Function8/1 -> Product54/2  "cos(3wt)"
  Math Function35/1 -> Add53/2  "Dab_3"
  Math Function24/1 -> Product48/2
  rx1/1 -> Product27/1, Product5/2, Product54/1, Product4/1, Product65/2, Product56/1, Product55/1  "rx"
  Trigonometric Function7/1 -> Product27/2  "sin(3wt)"
  Math Function45/1 -> Add53/1
  ex/1 -> Math Function24/1
  Add27/1 -> Math Function34/1, Product50/1  "ZAB"
  Product5/1 -> Add38/2  "r/2"
  Product62/1 -> Add38/1  "r*sin(3wt)/2"
  Constant24/1 -> Math Function45/2
  Product57/1 -> Trigonometric Function12/1, Product29/2, Trigonometric Function11/1
  Product63/1 -> Product3/2, Product1/2  "1/2"
  Constant/1 -> Product63/2
  Constant19/1 -> Product62/2, Product5/1  "2"
  Math Function39/1 -> Add35/1  "10_exp(-100Dab/r)"
  Product1/1 -> Product2/2, Add27/3  "z4/2"
  Product50/1 -> Product40/1  "Nab"
  Constant1/1 -> Product63/1
  In1/1 -> Add27/2  "z0 - z + delta"
  Product48/1 -> Product66/2
  Product55/1 -> Add38/4  "r*sin(wt)"
  Product54/1 -> Add21/1  "r*cos(3wt)"
  Product4/1 -> Add27/4  "r*sqrt(3)/2"
  Sqrt14/1 -> Product3/1, Product2/1  "sqrt(3)"
  Product3/1 -> Product46/2, Product4/2  "sqrt(3)/2"

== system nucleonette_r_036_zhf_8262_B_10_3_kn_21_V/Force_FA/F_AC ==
  In1 : Inport
  In2 : Inport  Port=2
  Add21 : Sum  Inputs=--
  Add27 : Sum  Inputs=-+++
  Add32 : Sum  Inputs=+++
  Add35 : Sum
  Add38 : Sum  Inputs=---+
  Add53 : Sum
  C_100_1 : Constant  Value=-100
  C_10_1 : Constant  Value=10
  C_10_11_2 : Constant  Value=1E-21
  Clock1 : Clock
  Constant : Constant
  Constant1 : Constant  Value=2
  Constant13 : Constant  Value=3
  Constant15 : Constant  Value=1.0E-3
  Constant19 : Constant  Value=2
  Constant24 : Constant  Value=3
  Constant26 : Constant  Value=3
  Math Function{17,24,34,36} (4 alike) : Math  Operator=square
  Math Function35 : Math  Operator=pow
  Math Function39 : Math  Operator=pow
  Math Function45 : Math  Operator=pow
  Nacx/Dacx : Scope
  Omega_w1 : Constant  Value=0.00003453723537
  Product{1..4,27,54..56,66} (9 alike) : Product  Inputs=**
  Product{29,46,50,57} (4 alike) : Product
  Product40 : Product  Inputs=*/
  Product48 : Product  Inputs=/**
  Product5 : Product  Inputs=/*
  Product62 : Product  Inputs=*/
  Product63 : Product  Inputs=/*
  Product65 : Product  Inputs=*/*
  Sqrt10 : Sqrt
  Sqrt14 : Sqrt
  Trigonometric Function11 : Trigonometry
  Trigonometric Function12 : Trigonometry  Operator=cos
  Trigonometric Function7 : Trigonometry
  Trigonometric Function8 : Trigonometry  Operator=cos
  ex : Constant  Value=1.602176565
  kACx : Constant  Value=66.535517341
  mFAx : Constant  Value=999.755388642
  rx1 : Constant  Value=0.36373
  Out1 : Outport
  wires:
  Add38/1 -> Math Function17/1  "YAC"
  Math Function36/1 -> Add32/2  "Xac_2"
  mFAx/1 -> Product48/1  "mx"
  Constant15/1 -> Math Function45/1
  C_100_1/1 -> Product65/3
  Sqrt14/1 -> Product3/1, Product2/1  "sqrt(3)"
  Product55/1 -> Add38/4  "r*sin(wt)"
  Product4/1 -> Add27/4  "r*sqrt(3)/2"
  Math Function39/1 -> Add35/1  "10_exp(-100Dac/r)"
  Constant1/1 -> Product63/1
  Product50/1 -> Product40/1  "Nac"
  Product54/1 -> Add21/1  "r*cos(3wt)"
  Product3/1 -> Product46/2, Product4/2  "sqrt(3)/2"
  Product48/1 -> Product66/2
  Product1/1 -> Product2/2, Add27/3  "z4/2"
  In1/1 -> Add27/2  "z0 - z + delta"
  Add21/1 -> Math Function36/1  "XAC"
  Trigonometric Function11/1 -> Product55/2  "sin(wt)"
  Add35/1 -> Product66/1
  Math Function35/1 -> Add53/2  "Dac_3"
  Trigonometric Function8/1 -> Product54/2  "cos(3wt)"
  Math Function24/1 -> Product48/2
  Product56/1 -> Add21/2  "r*cos(wt)"
  Trigonometric Function7/1 -> Product27/2  "sin(3wt)"
  Constant19/1 -> Product62/2, Product5/1  "2"
  Constant/1 -> Product63/2
  Product2/1 -> Add38/3  "z4*sqrt(3)/2"
  Trigonometric Function12/1 -> Product56/2  "cos(wt)"
  Clock1/1 -> Product57/1
  Constant26/1 -> Math Function35/2
  Product29/1 -> Trigonometric Function8/1, Trigonometric Function7/1
  Product46/1 -> Add27/1  "r*sin(3wt)*sqrt(3)/2"
  Product65/1 -> Math Function39/2
  C_10_1/1 -> Math Function39/1
  Constant24/1 -> Math Function45/2
  ex/1 -> Math Function24/1
  Product57/1 -> Trigonometric Function12/1, Product29/2, Trigonometric Function11/1
  Math Function34/1 -> Add32/3  "Zac_2"
  Product63/1 -> Product3/2, Product1/2  "1/2"
  Product5/1 -> Add38/2  "r/2"
  Add27/1 -> Math Function34/1, Product50/1  "ZAC"
  Omega_w1/1 -> Product57/2
  Constant13/1 -> Product29/1, Sqrt14/1
  Add32/1 -> Sqrt10/1  "Dac_2"
  Product40/1 -> Nacx/Dacx/1, Out1/1  "nac/dac"
  Product27/1 -> Product46/1, Product62/1  "r*sin(3wt)"
  Math Function45/1 -> Add53/1
  Product66/1 -> Product50/2  "kn_Dac"
  Product62/1 -> Add38/1  "r*sin(3wt)/2"
  kACx/1 -> Product48/3
  Add53/1 -> Product40/2  "Dac_B"
  rx1/1 -> Product27/1, Product5/2, Product54/1, Product4/1, Product65/2, Product56/1, Product55/1  "rx"
  Sqrt10/1 -> Product65/1, Math Function35/1  "Dac"
  C_10_11_2/1 -> Add35/2
  Math Function17/1 -> Add32/1  "Yac_2"
  In2/1 -> Product1/1  "z4"
